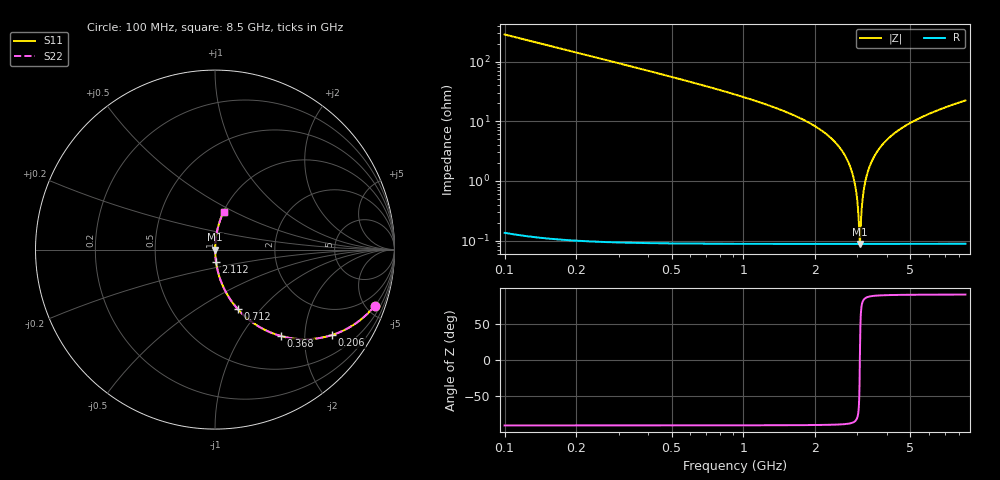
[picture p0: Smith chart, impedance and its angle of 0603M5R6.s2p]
! Created Wed Apr 18 15:56:47 2012
# hz S ma R 50
! 2 Port Network Data from SP1.SP block
! freq  magS11  angS11  magS21  angS21  magS12  angS12  magS22  angS22
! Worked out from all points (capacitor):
!   8401 points, 100 MHz to 8.5 GHz, reference 50 ohm
!   read as one part in series: C = 5.6 pF near 142 MHz
!   lowest |Z| = 88.1 mohm at 3.073 GHz (marker M1)
!   series resonance near 3.073 GHz, so ESL is about 480 pH
!   S11 on the Smith chart (normalised r, x): 100 MHz: 1.00, -5.68; 206 MHz: 1.00, -2.75; 368 MHz: 1.00, -1.52; 712 MHz: 1.00, -0.76; 2.112 GHz: 1.00, -0.14; 8.5 GHz: 1.00, +0.45
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1e8  0.9431 -19.4  0.3322 70.6  0.3322 70.6  0.9431 -19.4
2.06e8  0.8081 -36.0  0.5884 53.9  0.5884 53.9  0.8081 -36.0
3.68e8  0.6054 -52.7  0.7952 37.3  0.7952 37.3  0.6054 -52.7
7.12e8  0.3531 -69.2  0.9348 20.7  0.9348 20.7  0.3531 -69.2
1.5e9  0.1427 -81.4  0.9889 8.2  0.9889 8.2  0.1427 -81.4
2.112e9  0.07077 -85.2  0.9966 4.1  0.9966 4.1  0.07077 -85.2
2.618e9  0.02974 -86.6  0.9987 1.7  0.9987 1.7  0.02974 -86.6
2.782e9  0.01843 -86.2  0.999 1.1  0.999 1.1  0.01843 -86.2
2.9e9  0.01074 -84.7  0.9991 0.6  0.9991 0.6  0.01074 -84.7
2.979e9  0.0058 -80.9  0.9991 0.3  0.9991 0.3  0.0058 -80.9
3.047e9  0.001791 -60.5  0.9991 0.1  0.9991 0.1  0.001791 -60.5
3.073e9  0.00088 0.7  0.9991 -0.0  0.9991 -0.0  0.00088 0.7
3.097e9  0.001696 58.7  0.9991 -0.1  0.9991 -0.1  0.001696 58.7
3.148e9  0.004556 78.6  0.9991 -0.3  0.9991 -0.3  0.004556 78.6
3.201e9  0.00761 82.9  0.9991 -0.4  0.9991 -0.4  0.00761 82.9
3.281e9  0.01216 85.2  0.999 -0.7  0.999 -0.7  0.01216 85.2
3.389e9  0.01816 86.2  0.999 -1.0  0.999 -1.0  0.01816 86.2
3.743e9  0.03671 86.5  0.9984 -2.1  0.9984 -2.1  0.03671 86.5
4.3e9  0.06321 85.6  0.9971 -3.6  0.9971 -3.6  0.06321 85.6
5.7e9  0.1209 82.6  0.9918 -6.9  0.9918 -6.9  0.1209 82.6
7.1e9  0.1713 79.8  0.9843 -9.9  0.9843 -9.9  0.1713 79.8
8.5e9  0.2176 77.2  0.9752 -12.6  0.9752 -12.6  0.2176 77.2
